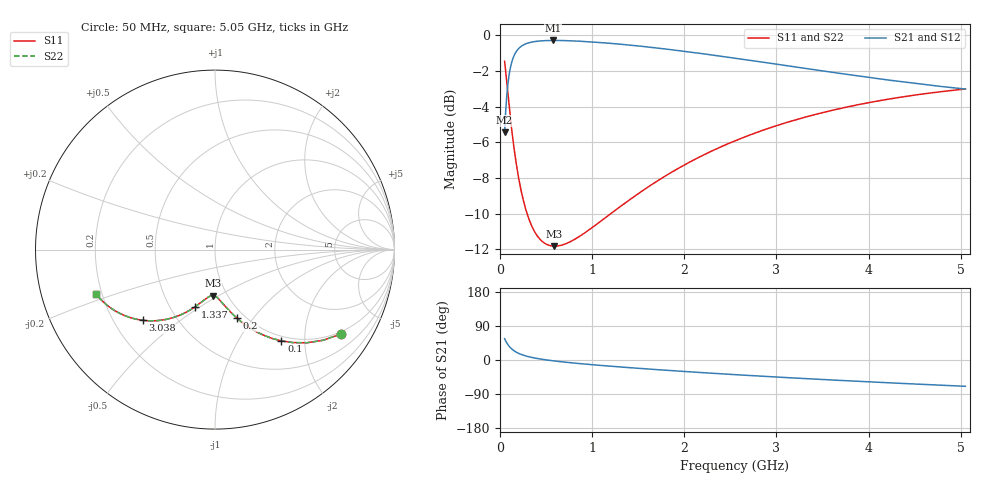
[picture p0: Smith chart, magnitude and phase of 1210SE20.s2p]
! AVX Thin Film Operation		Date: August 2001
! Description: Accu-P® Series, Thin Film, SMD, RF Capacitor
! Part Number: 12101J200FBT
! 50 MHz  -  5.05 GHz
! Serial Measurements
# mhz S db R 50
!	S11		S21		S12		S22
!	dB	Phase	dB	Phase	dB	Phase	dB	Phase
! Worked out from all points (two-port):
!   401 points, 50 MHz to 5.05 GHz, reference 50 ohm
!   highest |S21| = -0.30 dB at 575 MHz (marker M1); lowest = -5.4 dB at 50 MHz (marker M2)
!   |S21| within 3 dB of the highest: 75 MHz to end of sweep
!   lowest |S11| = -11.8 dB at 587.5 MHz (marker M3), VSWR 1.69, Z = 43 - j23.6 ohm
!   |S11| at or under -10 dB: 293.9 MHz to 1.202 GHz (907.9 MHz wide, 121 % of centre)
!   |S22| runs from -11.8 to -1.5 dB; largest |S21 - S12| = 0
!   S11 on the Smith chart (normalised r, x): 50 MHz: 0.92, -3.04; 100 MHz: 0.92, -1.55; 200 MHz: 0.92, -0.83; 1.337 GHz: 0.67, -0.48; 3.038 GHz: 0.32, -0.37; 5.05 GHz: 0.18, -0.18
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50  -1.46 -33.8  -5.45 56.2  -5.45 56.2  -1.46 -33.8
62.5  -2.09 -40.0  -4.19 50.0  -4.19 50.0  -2.09 -40.0
87.5  -3.40 -50.0  -2.66 40.0  -2.66 40.0  -3.40 -50.0
100  -4.03 -54.0  -2.19 36.0  -2.19 36.0  -4.03 -54.0
112.5  -4.64 -57.4  -1.83 32.6  -1.83 32.6  -4.64 -57.4
137.5  -5.75 -63.0  -1.35 27.0  -1.35 27.0  -5.75 -63.0
162.5  -6.72 -67.3  -1.04 22.7  -1.04 22.7  -6.72 -67.3
200  -7.94 -72.3  -0.76 17.7  -0.76 17.7  -7.94 -72.3
275  -9.68 -79.0  -0.50 11.0  -0.50 11.0  -9.68 -79.0
362.5  -10.89 -84.1  -0.37 5.9  -0.37 5.9  -10.89 -84.1
462.5  -11.57 -88.3  -0.32 1.6  -0.32 1.6  -11.57 -88.3
575  -11.82 -92.1  -0.30 -2.1  -0.30 -2.1  -11.82 -92.1
587.5  -11.82 -92.4  -0.30 -2.5  -0.30 -2.5  -11.82 -92.4
887.5  -11.19 -100.0  -0.34 -10.0  -0.34 -10.0  -11.19 -100.0
1337.5  -9.48 -109.0  -0.52 -19.0  -0.52 -19.0  -9.48 -109.0
1725  -8.11 -115.8  -0.73 -25.8  -0.73 -25.8  -8.11 -115.8
2125  -6.93 -122.2  -0.99 -32.3  -0.99 -32.3  -6.93 -122.2
2550  -5.92 -128.6  -1.29 -38.6  -1.29 -38.6  -5.92 -128.6
3037.5  -5.01 -135.4  -1.65 -45.5  -1.65 -45.5  -5.01 -135.4
3387.5  -4.49 -140.0  -1.92 -50.0  -1.92 -50.0  -4.49 -140.0
4225  -3.58 -150.2  -2.52 -60.2  -2.52 -60.2  -3.58 -150.2
5050  -3.02 -159.4  -3.02 -69.4  -3.02 -69.4  -3.02 -159.4
